(* Logix 5000 AddOnInstructionDefinition export SPEL_Above; software revision 30.01; part 8 of 9 *)

ADD_ON_INSTRUCTION SPEL_Speed   (* revision 1.0, vendor SEIKO EPSON CORP. *)
// Sets the arm speed setting of PTP motion.
VAR_OUTPUT
   InCycle : BOOL; {access Read Only, visible}
   Done : BOOL; {access Read Only, visible}
   Error : BOOL; {access Read Only, visible}
END_VAR
VAR_INPUT
   Start : BOOL; {required}
   Speed : INT; {required}
   ApproSpeed : INT; {required}
   DepartSpeed : INT; {required}
END_VAR
VAR_IN_OUT
   ExtInputs : AB:ETHERNET_MODULE_INT_128Bytes:I:0; {required}
   ExtOutputs : AB:ETHERNET_MODULE_INT_128Bytes:O:0; {required}
END_VAR
VAR_OUTPUT
   ErrCode1 : INT; {access Read Only, visible}
   ErrCode2 : INT; {access Read Only, visible}
END_VAR
VAR
   ExecSpeed : SPEL_ExecCmd := (MaxTime := 3000); {access None}
        .INCYCLE   // ExecInCycle
        .DONE   // ExecDone
        .ERROR   // ExecError
   OneShotStart : BOOL; {access None}
   StartCoil : BOOL; {access None}
   ExecTimeout : DINT; {access None}
END_VAR

ROUTINE Logic   (* ladder *)
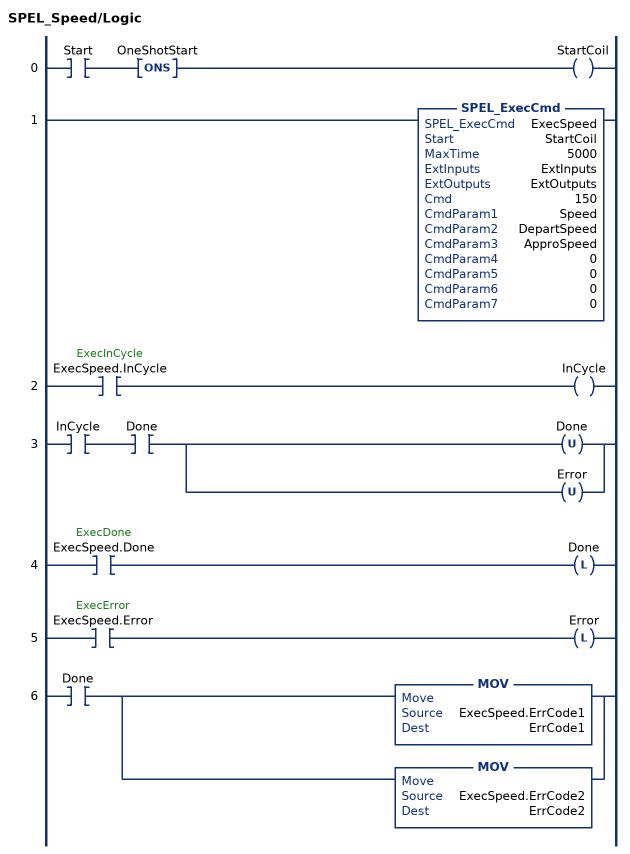
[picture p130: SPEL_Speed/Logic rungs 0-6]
   0: XIC(Start)ONS(OneShotStart)OTE(StartCoil);
   1: SPEL_ExecCmd(ExecSpeed,StartCoil,5000,ExtInputs,ExtOutputs,150,Speed,DepartSpeed,ApproSpeed,0,0,0,0);
   2: XIC(ExecSpeed.InCycle)OTE(InCycle);
   3: XIC(InCycle)XIC(Done)[OTU(Done) ,OTU(Error) ];
   4: XIC(ExecSpeed.Done)OTL(Done);
   5: XIC(ExecSpeed.Error)OTL(Error);
   6: XIC(Done)[MOV(ExecSpeed.ErrCode1,ErrCode1) ,MOV(ExecSpeed.ErrCode2,ErrCode2) ];
END_ROUTINE
END_ADD_ON_INSTRUCTION

ADD_ON_INSTRUCTION SPEL_SpeedS   (* revision 1.0, vendor SEIKO EPSON CORP. *)
// Sets the arm speed setting of CP motion. This will set the depart, and approach speed as well.
VAR_OUTPUT
   InCycle : BOOL; {access Read Only, visible}
   Done : BOOL; {access Read Only, visible}
   Error : BOOL; {access Read Only, visible}
END_VAR
VAR_INPUT
   Start : BOOL; {required}
   Speed : REAL; {required}
   ApproSpeed : REAL; {required}
   DepartSpeed : REAL; {required}
END_VAR
VAR_IN_OUT
   ExtInputs : AB:ETHERNET_MODULE_INT_128Bytes:I:0; {required}
   ExtOutputs : AB:ETHERNET_MODULE_INT_128Bytes:O:0; {required}
END_VAR
VAR_OUTPUT
   ErrCode1 : INT; {access Read Only, visible}
   ErrCode2 : INT; {access Read Only, visible}
END_VAR
VAR
   ExecSpeedS : SPEL_ExecCmd := (MaxTime := 3000); {access None}
   OneShotStart : BOOL; {access None}
   StartInit : BOOL; {access None}
   ApproachSp : DINT; {access None}
   Approachx1000 : DINT; {access None}
   DepartSp : DINT; {access None}
   Departx1000 : DINT; {access None}
   Approach_INTS : INT[2]; {access None}
   Depart_INTS : INT[2]; {access None}
   Speedx1000 : DINT; {access None}
   Speed_INTS : INT[2]; {access None}
   ExecTimeout : DINT; {access None}
END_VAR

ROUTINE Logic   (* ladder *)
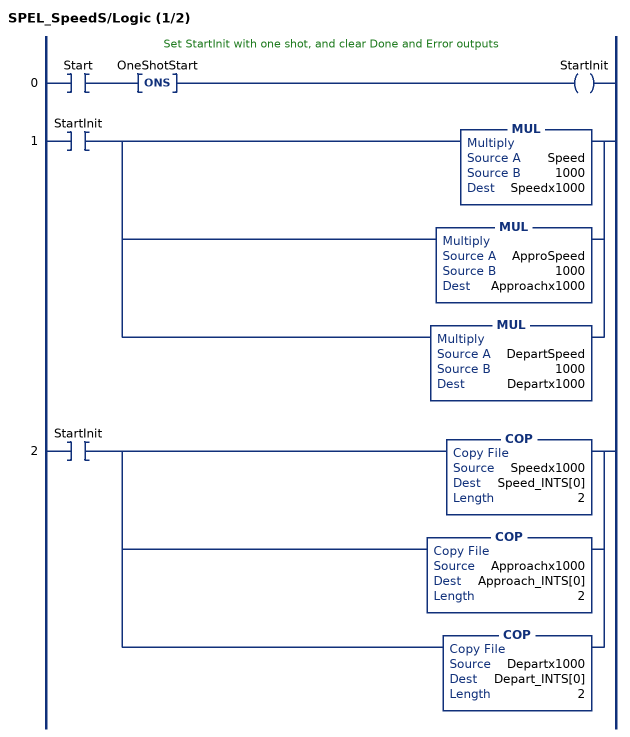
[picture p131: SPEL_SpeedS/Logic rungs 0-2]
   // Set StartInit with one shot, and clear Done and Error outputs
   0: XIC(Start)ONS(OneShotStart)OTE(StartInit);
   1: XIC(StartInit)[MUL(Speed,1000,Speedx1000) ,MUL(ApproSpeed,1000,Approachx1000) ,MUL(DepartSpeed,1000,Departx1000) ];
   2: XIC(StartInit)[COP(Speedx1000,Speed_INTS[0],2) ,COP(Approachx1000,Approach_INTS[0],2) ,COP(Departx1000,Depart_INTS[0],2) ];
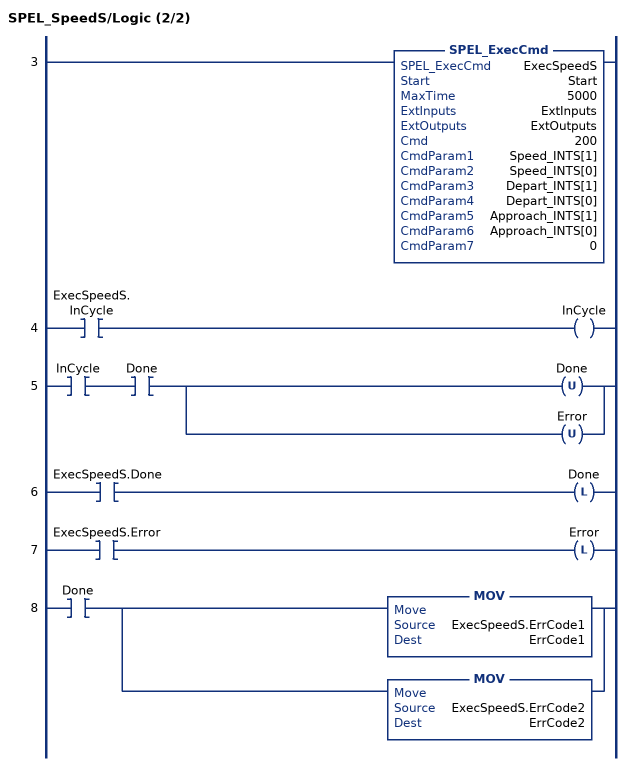
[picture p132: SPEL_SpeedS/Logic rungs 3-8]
   3: SPEL_ExecCmd(ExecSpeedS,Start,5000,ExtInputs,ExtOutputs,200,Speed_INTS[1],Speed_INTS[0],Depart_INTS[1],Depart_INTS[0],Approach_INTS[1],Approach_INTS[0],0);
   4: XIC(ExecSpeedS.InCycle)OTE(InCycle);
   5: XIC(InCycle)XIC(Done)[OTU(Done) ,OTU(Error) ];
   6: XIC(ExecSpeedS.Done)OTL(Done);
   7: XIC(ExecSpeedS.Error)OTL(Error);
   8: XIC(Done)[MOV(ExecSpeedS.ErrCode1,ErrCode1) ,MOV(ExecSpeedS.ErrCode2,ErrCode2) ];
END_ROUTINE
END_ADD_ON_INSTRUCTION

ADD_ON_INSTRUCTION SPEL_Sw   (* revision 1.0, vendor SEIKO EPSON CORP. *)
// Reads the status of an input bit.
VAR_OUTPUT
   InCycle : BOOL; {access Read Only, visible}
   Done : BOOL; {access Read Only, visible}
   Error : BOOL; {access Read Only, visible}
END_VAR
VAR_INPUT
   Start : BOOL; {access Read Only, required}
   Bit : INT; {required}
END_VAR
VAR_OUTPUT
   Status : INT; {access Read Only, visible}
END_VAR
VAR_IN_OUT
   ExtInputs : AB:ETHERNET_MODULE_INT_128Bytes:I:0; {required}
   ExtOutputs : AB:ETHERNET_MODULE_INT_128Bytes:O:0; {required}
END_VAR
VAR_OUTPUT
   ErrCode1 : INT; {access Read Only, visible}
   ErrCode2 : INT; {access Read Only, visible}
END_VAR
VAR
   ExecSw : SPEL_ExecCmd := (MaxTime := 3000); {access None}
        .INCYCLE   // ExecInCycle
        .DONE   // ExecDone
        .ERROR   // ExecError
   OneShotStart : BOOL; {access None}
   StartCoil : BOOL; {access None}
   ExecTimeout : DINT; {access None}
END_VAR

ROUTINE Logic   (* ladder *)
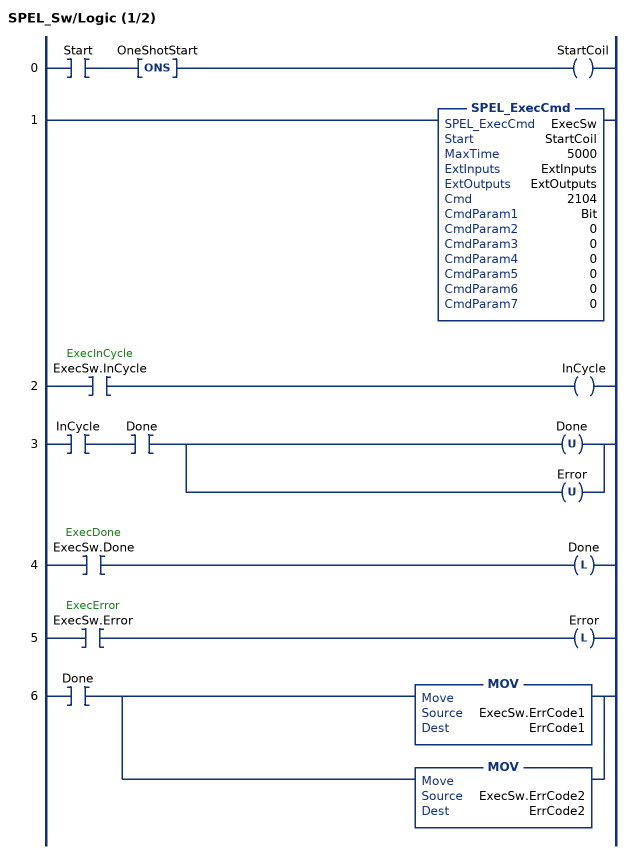
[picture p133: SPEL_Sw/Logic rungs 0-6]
   0: XIC(Start)ONS(OneShotStart)OTE(StartCoil);
   1: SPEL_ExecCmd(ExecSw,StartCoil,5000,ExtInputs,ExtOutputs,2104,Bit,0,0,0,0,0,0);
   2: XIC(ExecSw.InCycle)OTE(InCycle);
   3: XIC(InCycle)XIC(Done)[OTU(Done) ,OTU(Error) ];
   4: XIC(ExecSw.Done)OTL(Done);
   5: XIC(ExecSw.Error)OTL(Error);
   6: XIC(Done)[MOV(ExecSw.ErrCode1,ErrCode1) ,MOV(ExecSw.ErrCode2,ErrCode2) ];
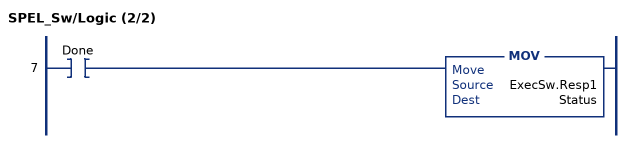
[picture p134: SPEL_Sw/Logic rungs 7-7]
   7: XIC(Done)MOV(ExecSw.Resp1,Status);
END_ROUTINE
END_ADD_ON_INSTRUCTION

ADD_ON_INSTRUCTION SPEL_TLSet   (* revision 1.2, vendor SEIKO EPSON CORP. *)
// Defines a tool coordinate system.
VAR_INPUT
   Start : BOOL; {access None, required}
END_VAR
VAR_OUTPUT
   InCycle : BOOL; {access Read Only, visible}
   Done : BOOL; {access Read Only, visible}
   Error : BOOL; {access Read Only, visible}
END_VAR
VAR_INPUT
   ToolNum : INT; {access None, required}
   Point : INT; {access None, required}
END_VAR
VAR_IN_OUT
   ExtInputs : AB:ETHERNET_MODULE_INT_128Bytes:I:0; {required}
   ExtOutputs : AB:ETHERNET_MODULE_INT_128Bytes:O:0; {required}
END_VAR
VAR_OUTPUT
   ErrCode1 : INT; {access Read Only, visible}
   ErrCode2 : INT; {access Read Only, visible}
END_VAR
VAR
   ExecTLSet : SPEL_ExecCmd := (MaxTime := 3000); {access None}
END_VAR

ROUTINE Logic   (* ladder *)
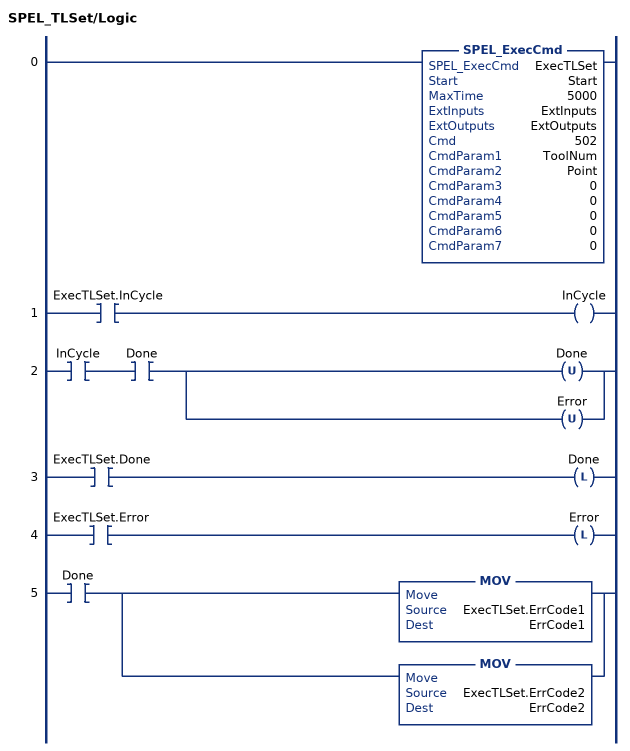
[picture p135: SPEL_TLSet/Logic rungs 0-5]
   0: SPEL_ExecCmd(ExecTLSet,Start,5000,ExtInputs,ExtOutputs,502,ToolNum,Point,0,0,0,0,0);
   1: XIC(ExecTLSet.InCycle)OTE(InCycle);
   2: XIC(InCycle)XIC(Done)[OTU(Done) ,OTU(Error) ];
   3: XIC(ExecTLSet.Done)OTL(Done);
   4: XIC(ExecTLSet.Error)OTL(Error);
   5: XIC(Done)[MOV(ExecTLSet.ErrCode1,ErrCode1) ,MOV(ExecTLSet.ErrCode2,ErrCode2) ];
END_ROUTINE
END_ADD_ON_INSTRUCTION

ADD_ON_INSTRUCTION SPEL_Teach   (* revision 1.0, vendor SEIKO EPSON CORP. *)
// Teaches the current position to the specified point.
VAR_OUTPUT
   InCycle : BOOL; {access Read Only, visible}
   Done : BOOL; {access Read Only, visible}
   Error : BOOL; {access Read Only, visible}
END_VAR
VAR_INPUT
   Start : BOOL; {required}
   Point : INT; {required}
END_VAR
VAR_IN_OUT
   ExtInputs : AB:ETHERNET_MODULE_INT_128Bytes:I:0; {required}
   ExtOutputs : AB:ETHERNET_MODULE_INT_128Bytes:O:0; {required}
END_VAR
VAR_OUTPUT
   ErrCode1 : INT; {access Read Only, visible}
   ErrCode2 : INT; {access Read Only, visible}
END_VAR
VAR
   ExecTeach : SPEL_ExecCmd := (MaxTime := 3000); {access None}
   OneShotStart : BOOL; {access None}
   StartCoil : BOOL; {access None}
   ExecTimeout : DINT; {access None}
END_VAR

ROUTINE Logic   (* ladder *)
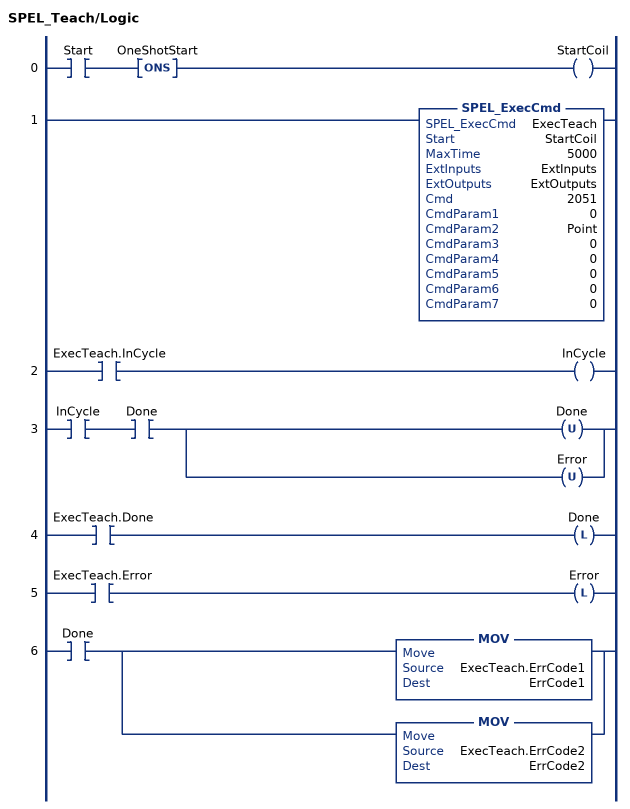
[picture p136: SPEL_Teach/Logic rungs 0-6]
   0: XIC(Start)ONS(OneShotStart)OTE(StartCoil);
   1: SPEL_ExecCmd(ExecTeach,StartCoil,5000,ExtInputs,ExtOutputs,2051,0,Point,0,0,0,0,0);
   2: XIC(ExecTeach.InCycle)OTE(InCycle);
   3: XIC(InCycle)XIC(Done)[OTU(Done) ,OTU(Error) ];
   4: XIC(ExecTeach.Done)OTL(Done);
   5: XIC(ExecTeach.Error)OTL(Error);
   6: XIC(Done)[MOV(ExecTeach.ErrCode1,ErrCode1) ,MOV(ExecTeach.ErrCode2,ErrCode2) ];
END_ROUTINE
END_ADD_ON_INSTRUCTION

ADD_ON_INSTRUCTION SPEL_ToolGet   (* revision 1.0, vendor SEIKO EPSON CORP. *)
// Aquires the tool selection status
VAR_OUTPUT
   InCycle : BOOL; {access Read Only, visible}
   Done : BOOL; {access Read Only, visible}
   Error : BOOL; {access Read Only, visible}
END_VAR
VAR_INPUT
   Start : BOOL; {required}
END_VAR
VAR_OUTPUT
   ToolNum : INT; {access Read Only, visible}
END_VAR
VAR_IN_OUT
   ExtInputs : AB:ETHERNET_MODULE_INT_128Bytes:I:0; {required}
   ExtOutputs : AB:ETHERNET_MODULE_INT_128Bytes:O:0; {required}
END_VAR
VAR_OUTPUT
   ErrCode1 : INT; {access Read Only, visible}
   ErrCode2 : INT; {access Read Only, visible}
END_VAR
VAR
   ExecToolGet : SPEL_ExecCmd := (MaxTime := 3000); {access None}
   OneShotStart : BOOL; {access None}
   StartCoil : BOOL; {access None}
   ExecTimeout : DINT; {access None}
END_VAR

ROUTINE Logic   (* ladder *)
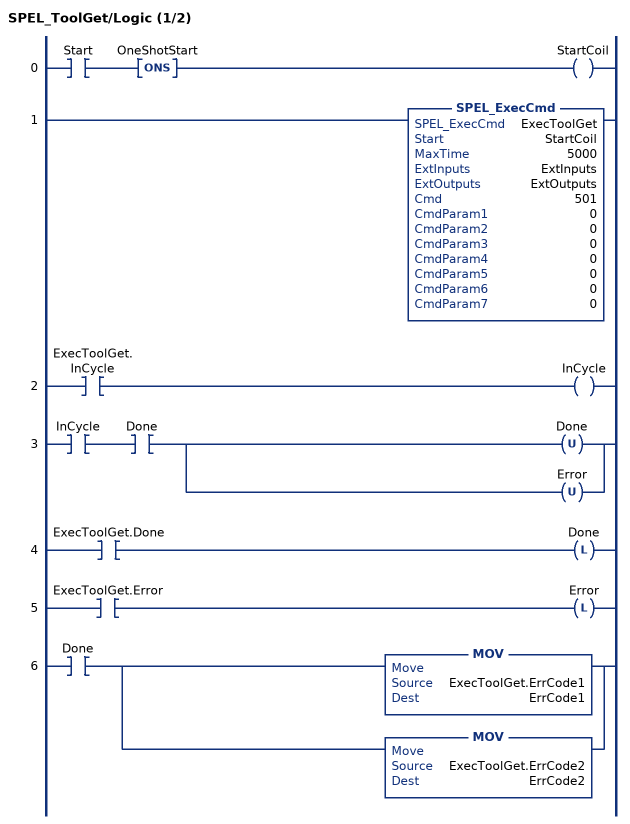
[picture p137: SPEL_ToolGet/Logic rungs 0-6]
   0: XIC(Start)ONS(OneShotStart)OTE(StartCoil);
   1: SPEL_ExecCmd(ExecToolGet,StartCoil,5000,ExtInputs,ExtOutputs,501,0,0,0,0,0,0,0);
   2: XIC(ExecToolGet.InCycle)OTE(InCycle);
   3: XIC(InCycle)XIC(Done)[OTU(Done) ,OTU(Error) ];
   4: XIC(ExecToolGet.Done)OTL(Done);
   5: XIC(ExecToolGet.Error)OTL(Error);
   6: XIC(Done)[MOV(ExecToolGet.ErrCode1,ErrCode1) ,MOV(ExecToolGet.ErrCode2,ErrCode2) ];
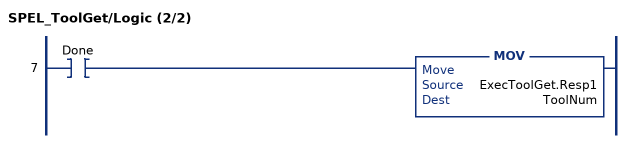
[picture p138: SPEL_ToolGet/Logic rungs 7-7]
   7: XIC(Done)MOV(ExecToolGet.Resp1,ToolNum);
END_ROUTINE
END_ADD_ON_INSTRUCTION

ADD_ON_INSTRUCTION SPEL_ToolSet   (* revision 1.0, vendor SEIKO EPSON CORP. *)
// Sets the tool selection status.
VAR_OUTPUT
   InCycle : BOOL; {access Read Only, visible}
   Done : BOOL; {access Read Only, visible}
   Error : BOOL; {access Read Only, visible}
END_VAR
VAR_INPUT
   Start : BOOL; {required}
   ToolNum : INT; {required}
END_VAR
VAR_IN_OUT
   ExtInputs : AB:ETHERNET_MODULE_INT_128Bytes:I:0; {required}
   ExtOutputs : AB:ETHERNET_MODULE_INT_128Bytes:O:0; {required}
END_VAR
VAR_OUTPUT
   ErrCode1 : INT; {access Read Only, visible}
   ErrCode2 : INT; {access Read Only, visible}
END_VAR
VAR
   ExecToolSet : SPEL_ExecCmd := (MaxTime := 3000); {access None}
   OneShotStart : BOOL; {access None}
   StartCoil : BOOL; {access None}
   ExecTimeout : DINT; {access None}
END_VAR

ROUTINE Logic   (* ladder *)
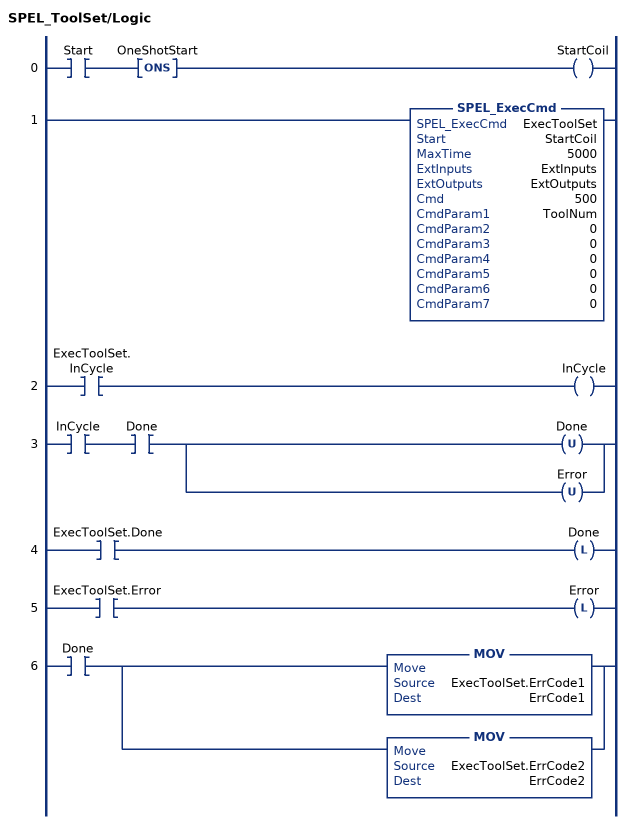
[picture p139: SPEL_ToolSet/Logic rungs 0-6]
   0: XIC(Start)ONS(OneShotStart)OTE(StartCoil);
   1: SPEL_ExecCmd(ExecToolSet,StartCoil,5000,ExtInputs,ExtOutputs,500,ToolNum,0,0,0,0,0,0);
   2: XIC(ExecToolSet.InCycle)OTE(InCycle);
   3: XIC(InCycle)XIC(Done)[OTU(Done) ,OTU(Error) ];
   4: XIC(ExecToolSet.Done)OTL(Done);
   5: XIC(ExecToolSet.Error)OTL(Error);
   6: XIC(Done)[MOV(ExecToolSet.ErrCode1,ErrCode1) ,MOV(ExecToolSet.ErrCode2,ErrCode2) ];
END_ROUTINE
END_ADD_ON_INSTRUCTION

ADD_ON_INSTRUCTION SPEL_WeightGet   (* revision 1.0, vendor SEIKO EPSON CORP. *)
// Gets the hand weight and arm length parameters.
VAR_OUTPUT
   InCycle : BOOL; {access Read Only, visible}
   Done : BOOL; {access Read Only, visible}
   Error : BOOL; {access Read Only, visible}
END_VAR
VAR_INPUT
   Start : BOOL; {required}
END_VAR
VAR_OUTPUT
   HandWeight : REAL; {visible}
   ArmLength : REAL; {visible}
END_VAR
VAR_IN_OUT
   ExtInputs : AB:ETHERNET_MODULE_INT_128Bytes:I:0; {required}
   ExtOutputs : AB:ETHERNET_MODULE_INT_128Bytes:O:0; {required}
END_VAR
VAR_OUTPUT
   ErrCode1 : DINT; {access Read Only, visible}
   ErrCode2 : DINT; {access Read Only, visible}
END_VAR
VAR
   ExecWeightGet : SPEL_ExecCmd := (MaxTime := 3000); {access None}
   HandWeightx1000 : DINT; {access None}
   HandWeight_INTS : INT[2]; {access None}
   ArmLengthx1000 : DINT; {access None}
   ArmLength_INTS : INT[2]; {access None}
   OneShotStart : BOOL; {access None}
   StartCoil : BOOL; {access None}
   ExecTimeout : DINT; {access None}
END_VAR

ROUTINE Logic   (* ladder *)
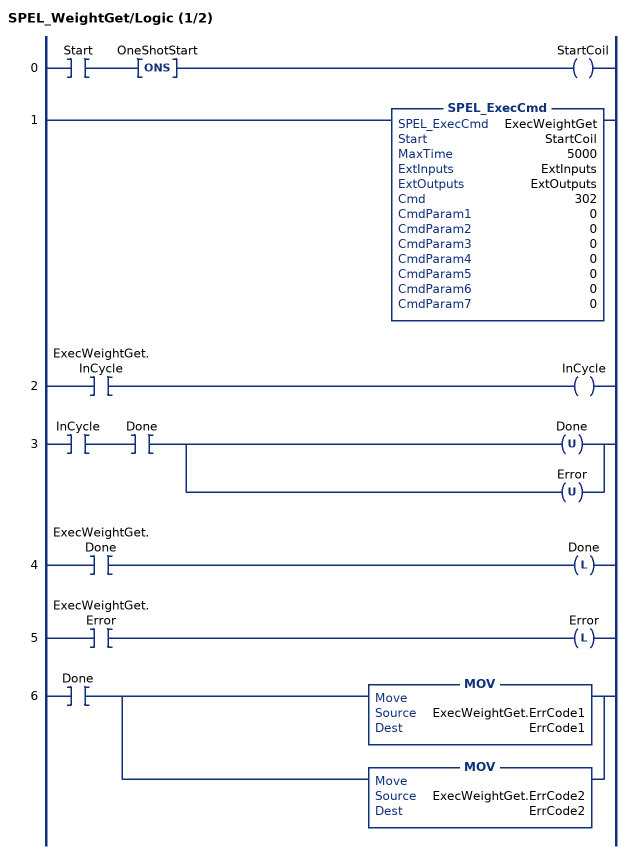
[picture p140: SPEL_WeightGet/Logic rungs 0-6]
   0: XIC(Start)ONS(OneShotStart)OTE(StartCoil);
   1: SPEL_ExecCmd(ExecWeightGet,StartCoil,5000,ExtInputs,ExtOutputs,302,0,0,0,0,0,0,0);
   2: XIC(ExecWeightGet.InCycle)OTE(InCycle);
   3: XIC(InCycle)XIC(Done)[OTU(Done) ,OTU(Error) ];
   4: XIC(ExecWeightGet.Done)OTL(Done);
   5: XIC(ExecWeightGet.Error)OTL(Error);
   6: XIC(Done)[MOV(ExecWeightGet.ErrCode1,ErrCode1) ,MOV(ExecWeightGet.ErrCode2,ErrCode2) ];
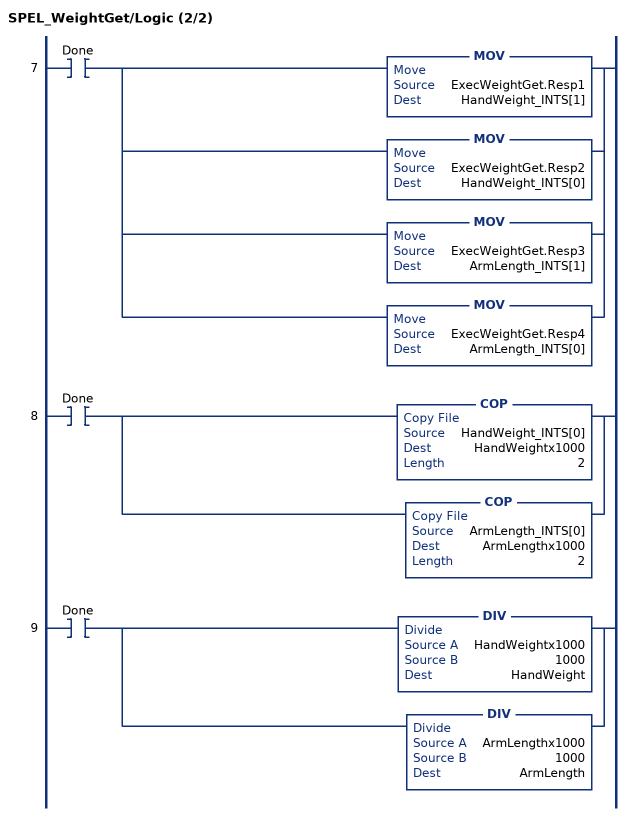
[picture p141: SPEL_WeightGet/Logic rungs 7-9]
   7: XIC(Done)[MOV(ExecWeightGet.Resp1,HandWeight_INTS[1]) ,MOV(ExecWeightGet.Resp2,HandWeight_INTS[0]) ,MOV(ExecWeightGet.Resp3,ArmLength_INTS[1]) ,MOV(ExecWeightGet.Resp4,ArmLength_INTS[0]) ];
   8: XIC(Done)[COP(HandWeight_INTS[0],HandWeightx1000,2) ,COP(ArmLength_INTS[0],ArmLengthx1000,2) ];
   9: XIC(Done)[DIV(HandWeightx1000,1000,HandWeight) ,DIV(ArmLengthx1000,1000,ArmLength) ];
END_ROUTINE
END_ADD_ON_INSTRUCTION

ADD_ON_INSTRUCTION SPEL_WeightSet   (* revision 1.0, vendor SEIKO EPSON CORP. *)
// Sets the weight parameter.
VAR_OUTPUT
   InCycle : BOOL; {access Read Only, visible}
   Done : BOOL; {access Read Only, visible}
   Error : BOOL; {access Read Only, visible}
END_VAR
VAR_INPUT
   Start : BOOL; {required}
   HandWeight : REAL; {required}
   ArmLength : REAL; {required}
END_VAR
VAR_IN_OUT
   ExtInputs : AB:ETHERNET_MODULE_INT_128Bytes:I:0; {required}
   ExtOutputs : AB:ETHERNET_MODULE_INT_128Bytes:O:0; {required}
END_VAR
VAR_OUTPUT
   ErrCode1 : INT; {access Read Only, visible}
   ErrCode2 : INT; {access Read Only, visible}
END_VAR
VAR
   ArmLengthx1000 : DINT; {access None}
   ArmLength_INTS : INT[2]; {access None}
   StartInit : BOOL; {access None}
   OneShotStart : BOOL; {access None}
   Weightx1000 : DINT; {access None}
   Weight_INTS : INT[2]; {access None}
   ExecWeightSet : SPEL_ExecCmd := (MaxTime := 3000); {access None}
   ExecTimeout : DINT; {access None}
END_VAR

ROUTINE Logic   (* ladder *)
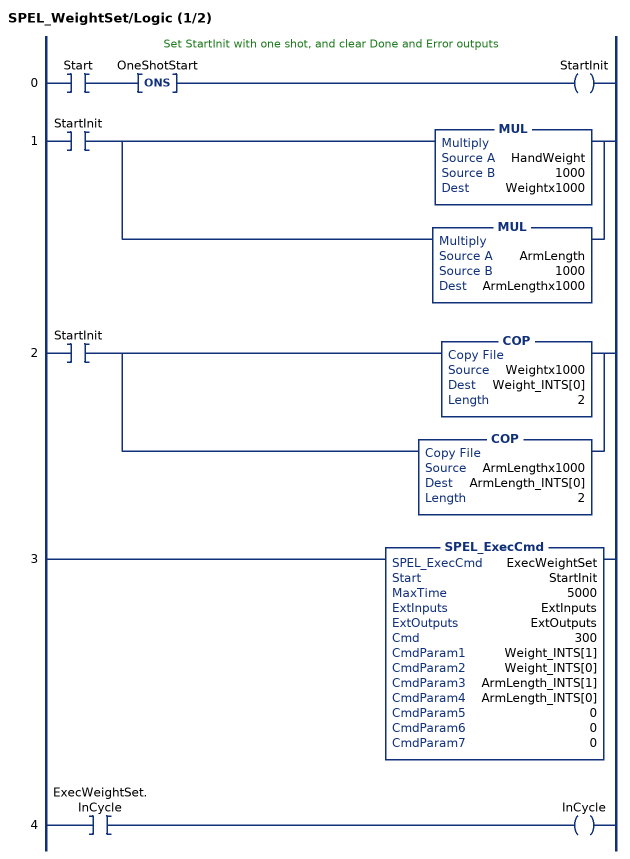
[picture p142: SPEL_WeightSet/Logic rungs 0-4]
   // Set StartInit with one shot, and clear Done and Error outputs
   0: XIC(Start)ONS(OneShotStart)OTE(StartInit);
   1: XIC(StartInit)[MUL(HandWeight,1000,Weightx1000) ,MUL(ArmLength,1000,ArmLengthx1000) ];
   2: XIC(StartInit)[COP(Weightx1000,Weight_INTS[0],2) ,COP(ArmLengthx1000,ArmLength_INTS[0],2) ];
   3: SPEL_ExecCmd(ExecWeightSet,StartInit,5000,ExtInputs,ExtOutputs,300,Weight_INTS[1],Weight_INTS[0],ArmLength_INTS[1],ArmLength_INTS[0],0,0,0);
   4: XIC(ExecWeightSet.InCycle)OTE(InCycle);
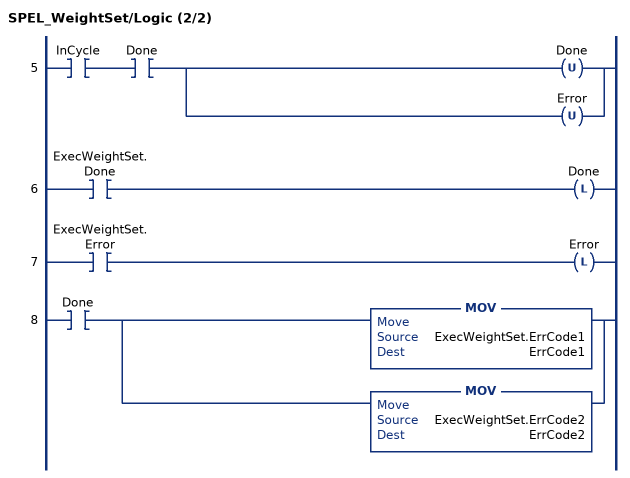
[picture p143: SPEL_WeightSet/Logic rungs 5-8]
   5: XIC(InCycle)XIC(Done)[OTU(Done) ,OTU(Error) ];
   6: XIC(ExecWeightSet.Done)OTL(Done);
   7: XIC(ExecWeightSet.Error)OTL(Error);
   8: XIC(Done)[MOV(ExecWeightSet.ErrCode1,ErrCode1) ,MOV(ExecWeightSet.ErrCode2,ErrCode2) ];
END_ROUTINE
END_ADD_ON_INSTRUCTION

ADD_ON_INSTRUCTION SPEL_XYLimGet   (* revision 1.0, vendor SEIKO EPSON CORP. *)
// Gets the setting value of the allowable motion
// area by specifying the lower and upper limit
// positions.
VAR_OUTPUT
   InCycle : BOOL; {access Read Only, visible}
   Done : BOOL; {access Read Only, visible}
   Error : BOOL; {access Read Only, visible}
END_VAR
VAR_INPUT
   Start : BOOL; {required}
END_VAR
VAR_OUTPUT
   XLower : REAL; {access Read Only, visible}
   XUpper : REAL; {access Read Only, visible}
   YLower : REAL; {access Read Only, visible}
   YUpper : REAL; {access Read Only, visible}
   ZLower : REAL; {access Read Only, visible}
   ZUpper : REAL; {access Read Only, visible}
END_VAR
VAR_IN_OUT
   ExtInputs : AB:ETHERNET_MODULE_INT_128Bytes:I:0; {required}
   ExtOutputs : AB:ETHERNET_MODULE_INT_128Bytes:O:0; {required}
END_VAR
VAR_OUTPUT
   ErrCode1 : INT; {access Read Only, visible}
   ErrCode2 : INT; {access Read Only, visible}
END_VAR
VAR
   ExecXYLimGetX : SPEL_ExecCmd := (MaxTime := 3000); {access None}
   lowerLimit_INTS : INT[2]; {access None}
   upperLimit_INTS : INT[2]; {access None}
   lowerLimitx1000 : DINT; {access None}
   upperLimitx1000 : DINT; {access None}
   StartInit : BOOL[32]; {access None}
   OneShotStart : BOOL[32]; {access None}
   ExecXYLimGetY : SPEL_ExecCmd := (MaxTime := 3000); {access None}
   ExecXYLimGetZ : SPEL_ExecCmd := (MaxTime := 3000); {access None}
   ExecTimeout : DINT; {access None}
END_VAR

ROUTINE Logic   (* ladder *)
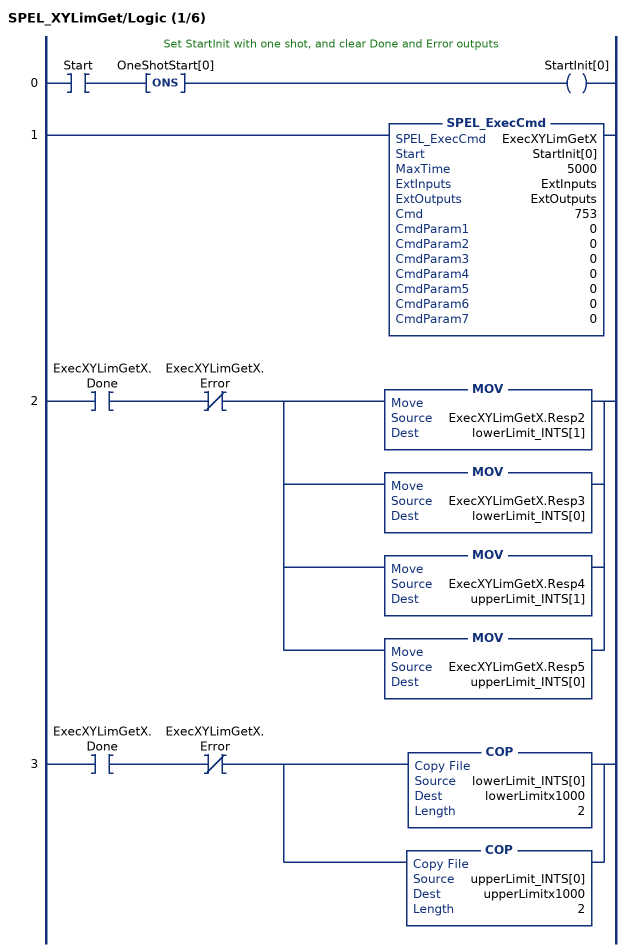
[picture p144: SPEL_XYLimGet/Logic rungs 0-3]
   // Set StartInit with one shot, and clear Done and Error outputs
   0: XIC(Start)ONS(OneShotStart[0])OTE(StartInit[0]);
   1: SPEL_ExecCmd(ExecXYLimGetX,StartInit[0],5000,ExtInputs,ExtOutputs,753,0,0,0,0,0,0,0);
   2: XIC(ExecXYLimGetX.Done)XIO(ExecXYLimGetX.Error)[MOV(ExecXYLimGetX.Resp2,lowerLimit_INTS[1]) ,MOV(ExecXYLimGetX.Resp3,lowerLimit_INTS[0]) ,MOV(ExecXYLimGetX.Resp4,upperLimit_INTS[1]) ,MOV(ExecXYLimGetX.Resp5,upperLimit_INTS[0]) ];
   3: XIC(ExecXYLimGetX.Done)XIO(ExecXYLimGetX.Error)[COP(lowerLimit_INTS[0],lowerLimitx1000,2) ,COP(upperLimit_INTS[0],upperLimitx1000,2) ];
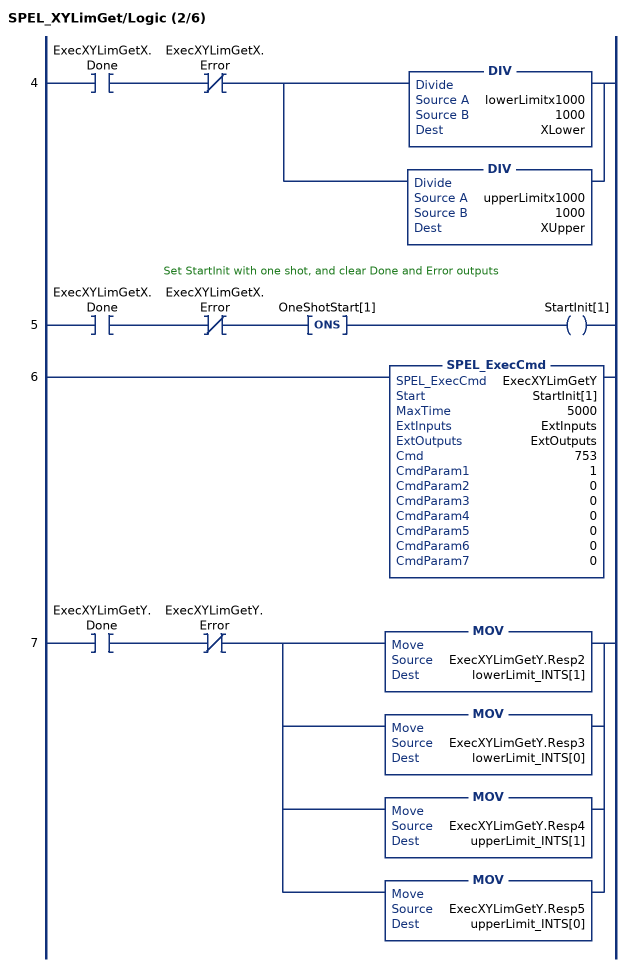
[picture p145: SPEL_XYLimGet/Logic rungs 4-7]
   4: XIC(ExecXYLimGetX.Done)XIO(ExecXYLimGetX.Error)[DIV(lowerLimitx1000,1000,XLower) ,DIV(upperLimitx1000,1000,XUpper) ];
   // Set StartInit with one shot, and clear Done and Error outputs
   5: XIC(ExecXYLimGetX.Done)XIO(ExecXYLimGetX.Error)ONS(OneShotStart[1])OTE(StartInit[1]);
   6: SPEL_ExecCmd(ExecXYLimGetY,StartInit[1],5000,ExtInputs,ExtOutputs,753,1,0,0,0,0,0,0);
   7: XIC(ExecXYLimGetY.Done)XIO(ExecXYLimGetY.Error)[MOV(ExecXYLimGetY.Resp2,lowerLimit_INTS[1]) ,MOV(ExecXYLimGetY.Resp3,lowerLimit_INTS[0]) ,MOV(ExecXYLimGetY.Resp4,upperLimit_INTS[1]) ,MOV(ExecXYLimGetY.Resp5,upperLimit_INTS[0]) ];
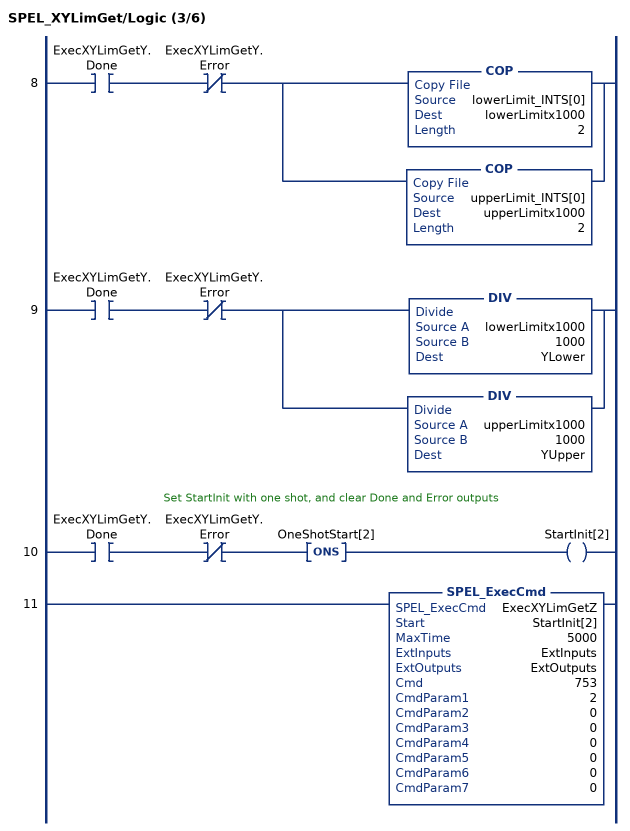
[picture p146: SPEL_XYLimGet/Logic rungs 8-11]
   8: XIC(ExecXYLimGetY.Done)XIO(ExecXYLimGetY.Error)[COP(lowerLimit_INTS[0],lowerLimitx1000,2) ,COP(upperLimit_INTS[0],upperLimitx1000,2) ];
   9: XIC(ExecXYLimGetY.Done)XIO(ExecXYLimGetY.Error)[DIV(lowerLimitx1000,1000,YLower) ,DIV(upperLimitx1000,1000,YUpper) ];
   // Set StartInit with one shot, and clear Done and Error outputs
   10: XIC(ExecXYLimGetY.Done)XIO(ExecXYLimGetY.Error)ONS(OneShotStart[2])OTE(StartInit[2]);
   11: SPEL_ExecCmd(ExecXYLimGetZ,StartInit[2],5000,ExtInputs,ExtOutputs,753,2,0,0,0,0,0,0);
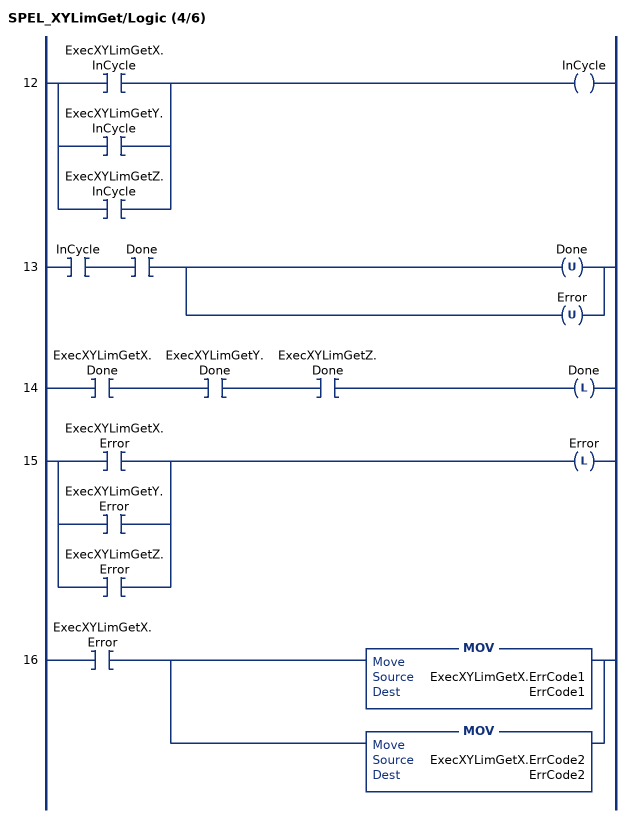
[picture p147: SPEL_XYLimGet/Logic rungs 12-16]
   12: [XIC(ExecXYLimGetX.InCycle) ,XIC(ExecXYLimGetY.InCycle) ,XIC(ExecXYLimGetZ.InCycle) ]OTE(InCycle);
   13: XIC(InCycle)XIC(Done)[OTU(Done) ,OTU(Error) ];
   14: XIC(ExecXYLimGetX.Done)XIC(ExecXYLimGetY.Done)XIC(ExecXYLimGetZ.Done)OTL(Done);
   15: [XIC(ExecXYLimGetX.Error) ,XIC(ExecXYLimGetY.Error) ,XIC(ExecXYLimGetZ.Error) ]OTL(Error);
   16: XIC(ExecXYLimGetX.Error)[MOV(ExecXYLimGetX.ErrCode1,ErrCode1) ,MOV(ExecXYLimGetX.ErrCode2,ErrCode2) ];
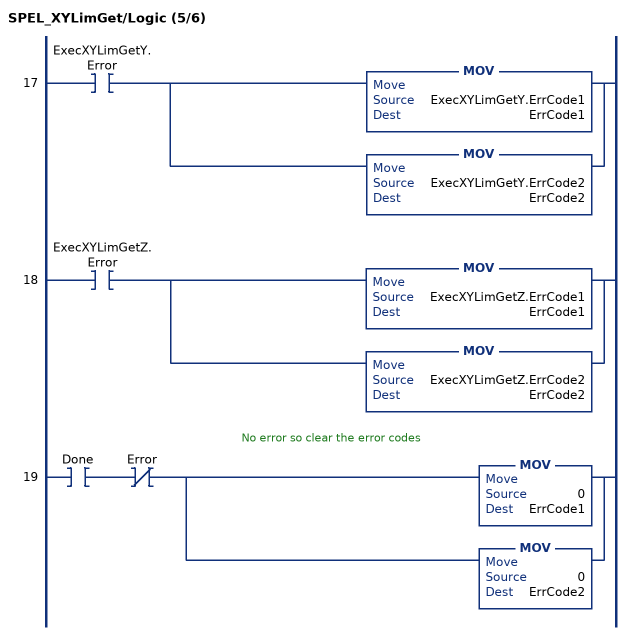
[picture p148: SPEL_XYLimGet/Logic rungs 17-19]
   17: XIC(ExecXYLimGetY.Error)[MOV(ExecXYLimGetY.ErrCode1,ErrCode1) ,MOV(ExecXYLimGetY.ErrCode2,ErrCode2) ];
   18: XIC(ExecXYLimGetZ.Error)[MOV(ExecXYLimGetZ.ErrCode1,ErrCode1) ,MOV(ExecXYLimGetZ.ErrCode2,ErrCode2) ];
   // No error so clear the error codes
   19: XIC(Done)XIO(Error)[MOV(0,ErrCode1) ,MOV(0,ErrCode2) ];
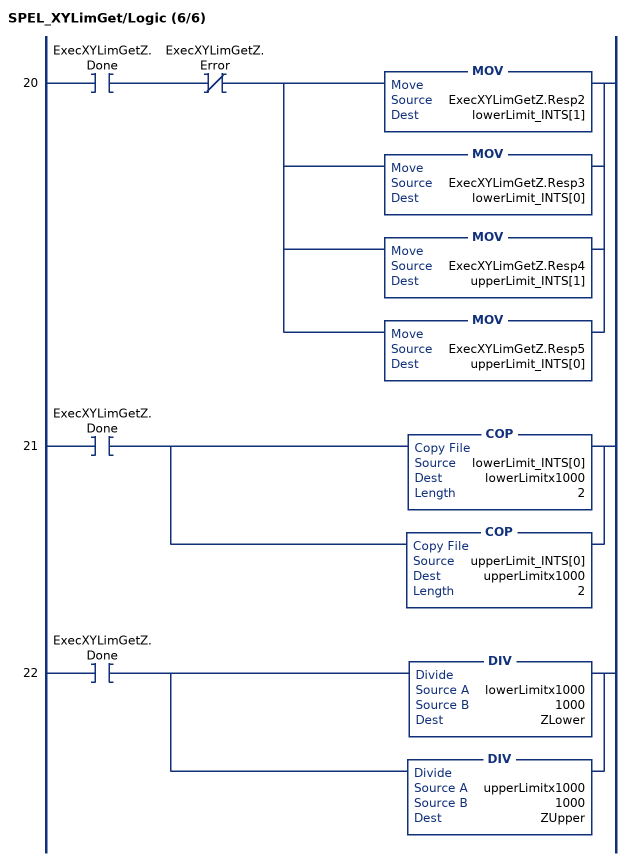
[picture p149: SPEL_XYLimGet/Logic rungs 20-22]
   20: XIC(ExecXYLimGetZ.Done)XIO(ExecXYLimGetZ.Error)[MOV(ExecXYLimGetZ.Resp2,lowerLimit_INTS[1]) ,MOV(ExecXYLimGetZ.Resp3,lowerLimit_INTS[0]) ,MOV(ExecXYLimGetZ.Resp4,upperLimit_INTS[1]) ,MOV(ExecXYLimGetZ.Resp5,upperLimit_INTS[0]) ];
   21: XIC(ExecXYLimGetZ.Done)[COP(lowerLimit_INTS[0],lowerLimitx1000,2) ,COP(upperLimit_INTS[0],upperLimitx1000,2) ];
   22: XIC(ExecXYLimGetZ.Done)[DIV(lowerLimitx1000,1000,ZLower) ,DIV(upperLimitx1000,1000,ZUpper) ];
END_ROUTINE
END_ADD_ON_INSTRUCTION
